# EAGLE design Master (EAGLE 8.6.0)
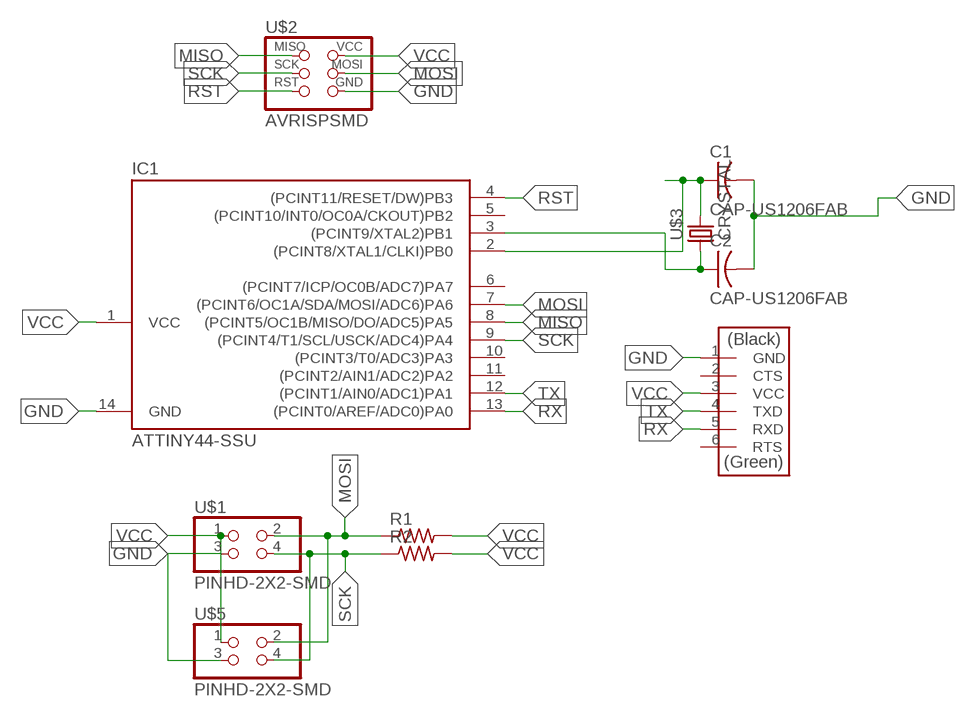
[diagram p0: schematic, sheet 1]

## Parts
C1  CAP-US1206FAB  [C1206FAB]
C2  CAP-US1206FAB  [C1206FAB]
IC1  ATTINY44-SSU  [SOIC14]
R1  RES-US1206FAB  [R1206FAB]
R2  RES-US1206FAB  [R1206FAB]
U$1  PINHD-2X2-SMD  [2X02SMD]
U$2  AVRISPSMD  [2X03SMD]
U$3  CRYSTAL  [2-SMD-5X3MM]
U$4  FTDI-SMD-HEADER  [1X06SMD]
U$5  PINHD-2X2-SMD  [2X02SMD]

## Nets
GND: C1.2 C2.2 IC1.14(GND) U$1.3 U$2.6(GND) U$4.1(GND) U$5.3
MISO: IC1.8((PCINT5/OC1B/MISO/DO/ADC5)PA5) U$2.1(MISO)
MOSI: IC1.7((PCINT6/OC1A/SDA/MOSI/ADC6)PA6) R1.1 U$1.2 U$2.4(MOSI) U$5.2
N$5: C2.1 IC1.3((PCINT9/XTAL2)PB1) U$3.P$1
N$6: C1.1 IC1.2((PCINT8/XTAL1/CLKI)PB0) U$3.P$2
RST: IC1.4((PCINT11/RESET/DW)PB3) U$2.5(RST)
RX: IC1.13((PCINT0/AREF/ADC0)PA0) U$4.5(RXD)
SCK: IC1.9((PCINT4/T1/SCL/USCK/ADC4)PA4) R2.1 U$1.4 U$2.3(SCK) U$5.4
TX: IC1.12((PCINT1/AIN0/ADC1)PA1) U$4.4(TXD)
VCC: IC1.1(VCC) R1.2 R2.2 U$1.1 U$2.2(VCC) U$4.3(VCC) U$5.1
Unconnected: IC1.5((PCINT10/INT0/OC0A/CKOUT)PB2) IC1.6((PCINT7/ICP/OC0B/ADC7)PA7) IC1.10((PCINT3/T0/ADC3)PA3) IC1.11((PCINT2/AIN1/ADC2)PA2) U$4.2(CTS) U$4.6(RTS)

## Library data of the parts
C1 C2 = fab:CAP-US
IC1 = fab:ATTINY44
R1 R2 = fab:RES-US: Resistor (US Symbol)
U$1 U$5 = fab:PINHD-2X2-SMD
U$2 = fab:AVRISP
U$3 = fab:CRYSTAL
U$4 = fab:FTDI-SMD-HEADER

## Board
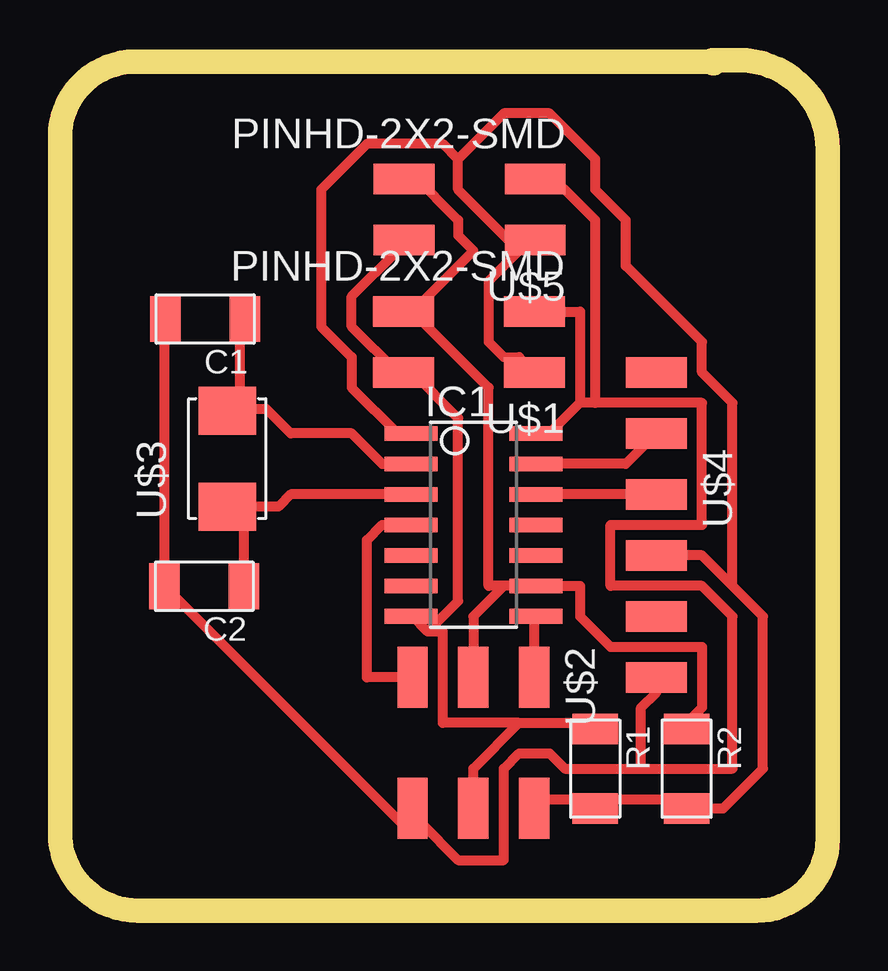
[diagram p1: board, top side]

Size 32.01 x 35.45 mm. Coordinates in mm from the lower left corner, seen from the top.
Outline: 27.18,35.38 3.13,35.38 arc90 0,32.25 0,3.26 arc90 3.26,0 29.02,0 arc90 32.01,2.99 32.01,31.71 arc90 28.27,35.45 27.25,35.45 arc90 27.18,35.38
Outline: 27.18,35.38 27.18,35.38
Outline: 27.18,35.38 arc90 27.25,35.31
Copper layers (1*16): Top 0.035mm / dielectric 1.5mm / Bottom 0.035mm
Design rules "default *": minimum track width 16mil, minimum drill 0.35mm, track to track 16mil, track to pad 16mil, pad to pad 16mil, via to via 16mil, smd to smd 16mil, copper to edge 16mil, drill to drill 16mil, minimum pad ring 10mil, minimum via ring 8mil, stop-mask expansion 4mil, vias tented up to drill 0mil, thermal gap 10mil

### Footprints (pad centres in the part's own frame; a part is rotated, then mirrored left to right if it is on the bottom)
C1206FAB = smd 1.27 x 1.905: 1 -1.651,0; 2 1.651,0
SOIC14 = smd 0.61 x 2.21: 1 -3.81,-2.603; 2 -2.54,-2.603; 3 -1.27,-2.603; 4 0,-2.603; 5 1.27,-2.603; 6 2.54,-2.603; 7 3.81,-2.603; 8 3.81,2.603; 9 2.54,2.603; 10 1.27,2.603; 11 0,2.603; 12 -1.27,2.603; 13 -2.54,2.603; 14 -3.81,2.603
R1206FAB = smd 1.27 x 1.905: 1 -1.651,0; 2 1.651,0
2X02SMD = smd 2.54 x 1.27: 1 -2.54,1.27; 2 2.92,1.27; 3 -2.54,-1.27; 4 2.92,-1.27
2X03SMD = smd 2.54 x 1.27: 1 -2.54,2.54; 2 2.92,2.54; 3 -2.54,0; 4 2.92,0; 5 -2.54,-2.54; 6 2.92,-2.54
2-SMD-5X3MM = smd 2 x 2.4: P$1 -2,0; P$2 2,0
1X06SMD = smd 2.54 x 1.27: 1 0,6.35; 2 0,3.81; 3 0,1.27; 4 0,-1.27; 5 0,-3.81; 6 0,-6.35

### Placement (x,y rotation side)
C1  6.05,24.66 180 top
C2  6.01,13.52 180 top
IC1  17.24,16.08 270 top
R1  22.32,5.92 270 top
R2  26.13,5.92 270 top
U$1  17.24,23.7 180 top
U$2  17.24,7.19 270 top
U$3  6.97,18.84 90 top
U$4  24.86,16.08 180 top
U$5  17.27,29.21 180 top

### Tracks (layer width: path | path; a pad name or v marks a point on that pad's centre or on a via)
GND
  Top 0.406: 21.68,21.16 20.41,19.89 IC1.14 | 21.68,21.16 21.68,24.97 U$1.3 | 14.7,4.65 U$2.6 14.7,4.01 15.03,3.69 | U$4.1 24.86,9.09 24.22,8.46 24.22,5.92 | 24.22,5.92 21.05,5.92 20.41,6.55 19.14,6.55 18.51,5.92 18.51,2.11 16.6,2.11 15.03,3.69 | 22.32,21.16 26.76,21.16 26.76,16.08 22.95,16.08 22.95,13.54 26.76,13.54 28.03,12.27 28.03,5.92 24.22,5.92 | 22.32,21.16 21.68,21.16 | 22.32,21.16 22.32,28.78 21.05,30.05 20.41,30.05 U$5.3 | C1.2 4.36,24.62 C2.2 14.2,3.69 15.03,3.69
MISO
  Top 0.406: U$2.1 19.78,12.27 IC1.8
MOSI
  Top 0.406: 19.14,7.82 22.32,7.82 R1.1 | 19.14,7.82 17.24,5.92 U$2.4 | 15.33,11.63 14.7,12.27 IC1.7 | 15.33,11.63 15.97,11.63 15.97,7.82 19.14,7.82 | 15.33,11.63 16.6,12.9 16.6,20.52 14.7,22.43 U$1.2 14.06,22.43 12.16,24.33 12.16,25.6 14.06,27.51 U$5.2
N$5
  Top 0.406: IC1.3 9.62,17.35 9.11,16.84 U$3.P$1 7.66,16.16 C2.1
N$6
  Top 0.406: IC1.2 13.43,18.62 12.16,19.89 9.62,19.89 8.61,20.9 7.98,20.9 7.92,20.84 7.49,20.84 | 7.49,20.84 U$3.P$2 | C1.1 7.49,24.45 7.49,20.84
RST
  Top 0.406: IC1.4 13.43,16.08 12.79,15.44 12.79,9.73 U$2.5
RX
  Top 0.406: IC1.13 23.59,18.62 U$4.5
SCK
  Top 0.406: R2.1 26.13,7.82 26.76,8.46 26.76,11 22.95,11 21.68,12.27 21.68,13.54 IC1.9 18.51,13.54 | 18.51,13.54 17.87,13.54 17.87,21.79 14.7,24.97 | U$2.3 17.24,12.27 18.51,13.54 | 14.7,24.97 17.24,27.51 16.6,28.14 16.6,28.78 14.7,30.68 U$5.4 | 14.7,24.97 U$1.4
TX
  Top 0.406: U$4.4 IC1.12
VCC
  Top 0.406: U$1.1 19.14,23.06 18.51,23.06 17.87,23.7 17.87,26.24 19.14,27.51 | IC1.1 14.06,19.89 12.16,21.79 12.16,23.06 10.89,24.33 10.89,30.05 12.79,31.95 15.97,31.95 16.6,31.32 | 19.14,27.51 19.78,28.14 U$5.1 19.14,27.51 | 16.6,31.32 16.6,30.05 19.14,27.51 | 22.32,4.65 19.78,4.65 U$2.2 | 22.32,4.65 26.13,4.65 R2.2 | 22.32,4.65 R1.2 | U$4.3 26.76,14.81 28.03,13.54 | 28.03,13.54 29.3,12.27 29.3,5.92 27.65,4.27 R2.2 | 26.13,4.01 R2.2 | 16.6,31.32 18.51,33.22 20.41,33.22 22.32,31.32 22.32,30.05 23.59,28.78 23.59,26.87 26.76,23.7 26.76,22.43 28.03,21.16 28.03,13.54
